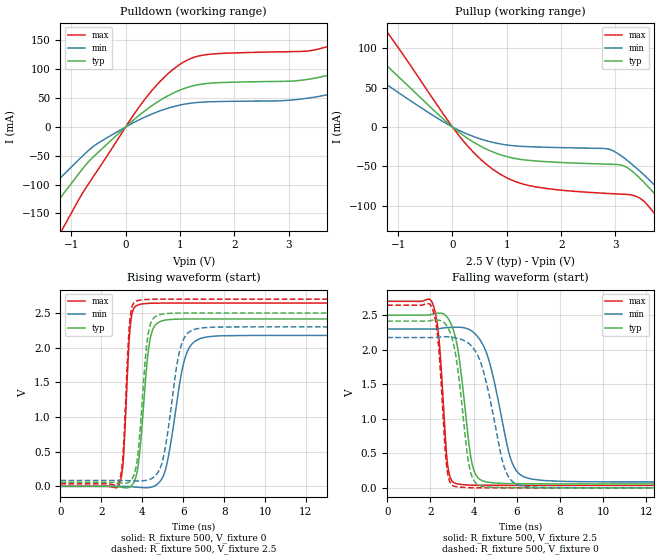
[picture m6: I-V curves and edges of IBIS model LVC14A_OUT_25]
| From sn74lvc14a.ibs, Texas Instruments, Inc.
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[Model]   LVC14A_OUT_25
Model_type  Output
Vref =   0
Rref =   500
Cref =   30p
Vmeas =   1.25
| variable   typ   min   max
C_comp   8.07pF   4.04pF   13.60pF
| C_pullup   6.98pF   4.04pF   8.24pF
| C_pulldown   9.17pF   4.37pF   13.60pF
[Temperature Range]   40   100   -40
| Ambient temperature   25   85   -40
[Voltage range]   2.5   2.3   2.7
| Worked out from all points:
|   slope of the pulldown table from 0 to 0.375 V, typ, clamps not added: 12.7 ohm
|   slope of the pullup table from 0 to 0.375 V, typ, clamps not added: 20 ohm
|   rising waveform, R_fixture 500, V_fixture 0: 20-80 % time 415ps typ, 712ps min, 257ps max; typ from 0 V to 2.41 V
|   falling waveform, R_fixture 500, V_fixture 2.5: 20-80 % time 558ps typ, 921ps min, 336ps max; typ from 2.5 V to 0.057 V
|   rising waveform, R_fixture 500, V_fixture 2.5: 20-80 % time 392ps typ, 651ps min, 252ps max; typ from 0.057 V to 2.5 V
|   falling waveform, R_fixture 500, V_fixture 0: 20-80 % time 545ps typ, 896ps min, 330ps max; typ from 2.41 V to 0 V
[Pulldown]
| LVC14A_OUT_25
|   Voltage   I(typ)   I(min)   I(max)
-5.5V     -601.9mA   -483.7mA   -770.2mA
-2.12V    -234.1mA   -175.5mA   -328.1mA
-1.58V    -169.3mA   -124.4mA   -246.1mA
-1.15V    -116.5mA   -83.59mA   -175.1mA
-565mV    -49.19mA   -31.73mA   -81.94mA
365mV     28.75mA    17.58mA    49.46mA
1.32V     73.05mA    42.4mA     122.5mA
4V        96.78mA    61.72mA    149.2mA
4.6V      117.3mA    77.78mA    177.9mA
5.77V     171.8mA    120.4mA    253.2mA
7.055V    245.3mA    179.5mA    351.5mA
11V       504.9mA    394.6mA    686.5mA
[Pullup]
| LVC14A_OUT_25
|   Voltage   I(typ)   I(min)   I(max)
-5.5V     363.4mA    279.9mA    508.8mA
-2.6V     169.4mA    122.6mA    251.6mA
-1.815V   117.7mA    83.03mA    179.1mA
-1.37V    88.47mA    61.37mA    136.9mA
170mV     -9.222mA   -5.867mA   -15.32mA
760mV     -32.2mA    -19.89mA   -54.58mA
2.88V     -47.3mA    -28.27mA   -84.56mA
3.45V     -65.22mA   -56.26mA   -90.57mA
3.915V    -100.8mA   -87.46mA   -129mA
4.185V    -124.1mA   -107.2mA   -157.5mA
4.495V    -152.3mA   -130.9mA   -192.5mA
11V       -836.4mA   -705.6mA   -1.028A
[Ramp]
| LVC14A_OUT_25
| variable   typ   min   max
dV/dt_r   1.46/4.27E-10   1.32/7.24E-10   1.60/2.71E-10
dV/dt_f   1.48/5.70E-10   1.34/9.39E-10   1.62/3.46E-10
R_load = 500
[Rising Waveform]
| LVC14A_OUT_25
R_fixture =   500
C_fixture =   0
L_fixture =   0
V_fixture =   0
V_fixture_min = 0
V_fixture_max = 0
|   Time   V(typ)   V(min)   V(max)
0s        177.7pV    3.876nV    17.91pV
2.87ns    -8.589mV   416.7uV    27.09mV
3.07ns    -17.72mV   -168.7uV   374.8mV
3.435ns   143.3uV    -5.649mV   2.364V
3.975ns   826.3mV    -17.77mV   2.63V
4.585ns   2.305V     2.55mV     2.641V
5.175ns   2.4V       284.8mV    2.643V
6.135ns   2.413V     1.892V     2.643V
7.165ns   2.414V     2.155V     2.644V
50ns      2.414V     2.176V     2.644V
[Falling Waveform]
| LVC14A_OUT_25
R_fixture =   500
C_fixture =   0
L_fixture =   0
V_fixture =   2.5
V_fixture_min = 2.3
V_fixture_max = 2.7
|   Time   V(typ)   V(min)   V(max)
0s        2.5V       2.3V       2.7V
2.115ns   2.517V     2.299V     2.659V
2.405ns   2.529V     2.304V     2.133V
2.815ns   2.455V     2.321V     301mV
3.325ns   1.895V     2.325V     54.15mV
4.115ns   185.9mV    2.216V     37.69mV
4.73ns    79.83mV    1.828V     36.25mV
5.79ns    60.72mV    361.3mV    35.96mV
6.8ns     58.03mV    122.2mV    35.94mV
50ns      57.33mV    84.96mV    35.94mV
[Rising Waveform]
| LVC14A_OUT_25
R_fixture =   500
C_fixture =   0
L_fixture =   0
V_fixture =   2.5
V_fixture_min = 2.3
V_fixture_max = 2.7
|   Time   V(typ)   V(min)   V(max)
0s        57.33mV    84.96mV    35.94mV
2.85ns    50.46mV    85.17mV    64.64mV
3.055ns   44.8mV     84.59mV    436.1mV
3.41ns    74.2mV     80.55mV    2.441V
3.9ns     835mV      78.13mV    2.686V
4.475ns   2.393V     114.9mV    2.698V
5.035ns   2.486V     421.3mV    2.7V
5.905ns   2.499V     2.037V     2.7V
6.8ns     2.5V       2.28V      2.7V
50ns      2.5V       2.3V       2.7V
[Falling Waveform]
| LVC14A_OUT_25
R_fixture =   500
C_fixture =   0
L_fixture =   0
V_fixture =   0
V_fixture_min = 0
V_fixture_max = 0
|   Time   V(typ)   V(min)   V(max)
0s        2.414V     2.176V     2.644V
2.095ns   2.426V     2.175V     2.594V
2.365ns   2.427V     2.179V     2.103V
2.77ns    2.341V     2.187V     269.1mV
3.185ns   1.9V       2.169V     17.49mV
3.735ns   431.2mV    2.101V     3.612mV
3.99ns    121.3mV    2.022V     1.677mV
5.455ns   2.668mV    271.4mV    26.23uV
6.32ns    642.5uV    21.63mV    2.832uV
50ns      3.253nV    -2.057nV   513.6pV
